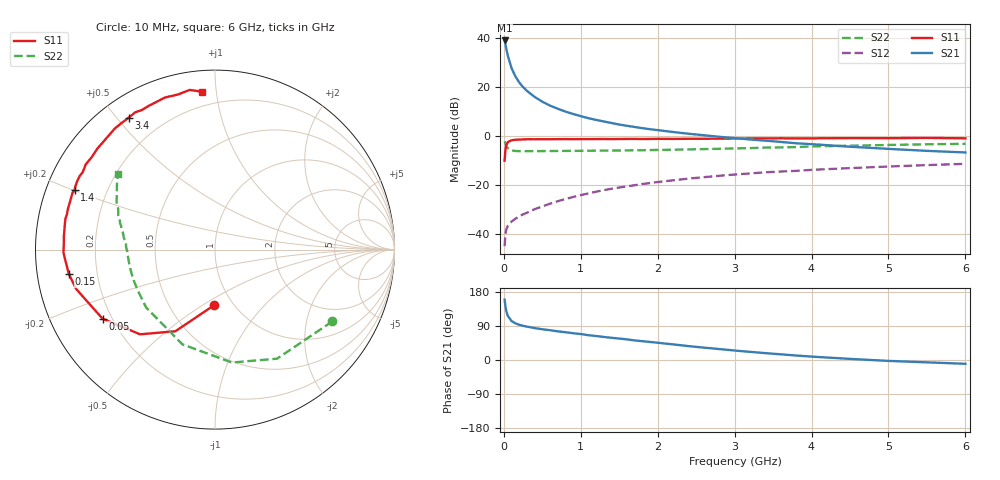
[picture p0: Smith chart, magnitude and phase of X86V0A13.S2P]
! SIEMENS Small Signal Semiconductors
! BFP136W
! Si NPN RF Bipolar Junction Transistor in SOT343
! VCE = 6 V  IC = 130 mA
! Common Emitter S-Parameters:  September  1994
# GHz  S  MA  R  50
!  f  S11  S21  S12  S22
! GHz  MAG  ANG  MAG  ANG  MAG  ANG  MAG  ANG
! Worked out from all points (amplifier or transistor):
!   40 points, 10 MHz to 6 GHz, reference 50 ohm
!   highest |S21| = 38.8 dB at 10 MHz (marker M1)
!   |S21| within 3 dB of that: start of sweep to 29.86 MHz
!   unconditionally stable (mu >= 1): 535 MHz to 2.975 GHz
!   at 200 MHz: K = 0.69, MSG = 27.2 dB, |S12| = -32.8 dB
!   at 1.5 GHz: K = 1.10, MAG = 10.9 dB, |S12| = -21.1 dB
!   at 6 GHz: K = 0.97, MSG = 2.3 dB, |S12| = -11.5 dB
!   S11 on the Smith chart (normalised r, x): 10 MHz: 0.82, -0.56; 50 MHz: 0.16, -0.28; 150 MHz: 0.10, -0.08; 1.4 GHz: 0.08, +0.20; 3.4 GHz: 0.08, +0.54; 6 GHz: 0.12, +0.92
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0.01  0.3088 -90.6  87.08 159.4  0.0056 68.4  0.7665 -31.5
0.02  0.5057 -115.9  73.64 142.4  0.0096 55.5  0.6991 -60.4
0.03  0.6301 -131.5  61.5 130.6  0.012 48.5  0.6362 -81.5
0.05  0.7354 -148.4  43.38 116.8  0.0145 38.9  0.5581 -109.0
0.1  0.8042 -164.2  23.79 102.8  0.0177 37.1  0.5012 -139.9
0.15  0.8254 -170.5  16.17 96.7  0.0203 40.0  0.4868 -152.5
0.2  0.8312 -173.9  12.15 92.9  0.0229 41.8  0.4842 -159.2
0.25  0.8386 -176.8  9.796 90.1  0.0249 44.4  0.4838 -163.6
0.3  0.8444 -178.9  8.193 88.1  0.0269 46.9  0.4831 -166.5
0.4  0.8429 177.5  6.168 84.3  0.0317 51.0  0.4841 -170.5
0.5  0.8454 174.8  4.92 81.1  0.0362 54.1  0.4853 -173.2
0.6  0.8462 172.7  4.103 78.6  0.041 55.9  0.486 -175.0
0.7  0.8486 170.2  3.54 75.6  0.0461 57.7  0.4875 -176.3
0.9  0.8479 166.6  2.769 70.7  0.0562 59.0  0.4894 -178.9
1.1  0.8504 162.1  2.266 65.4  0.0666 59.8  0.4928 179.5
1.4  0.8503 157.0  1.808 58.6  0.0828 59.5  0.4962 177.0
2.2  0.8585 143.2  1.187 41.2  0.1232 54.4  0.5161 171.0
3.2  0.8765 126.3  0.836 21.5  0.17 45.2  0.5576 162.4
3.4  0.8787 123.2  0.791 18.1  0.1793 43.1  0.5709 160.7
4.5  0.8918 108.2  0.595 2.9  0.2181 33.8  0.6241 151.3
5.5  0.9007 99.0  0.49 -6.2  0.2512 25.5  0.667 144.9
6  0.8824 94.6  0.455 -10.0  0.2669 21.2  0.6825 142.0
